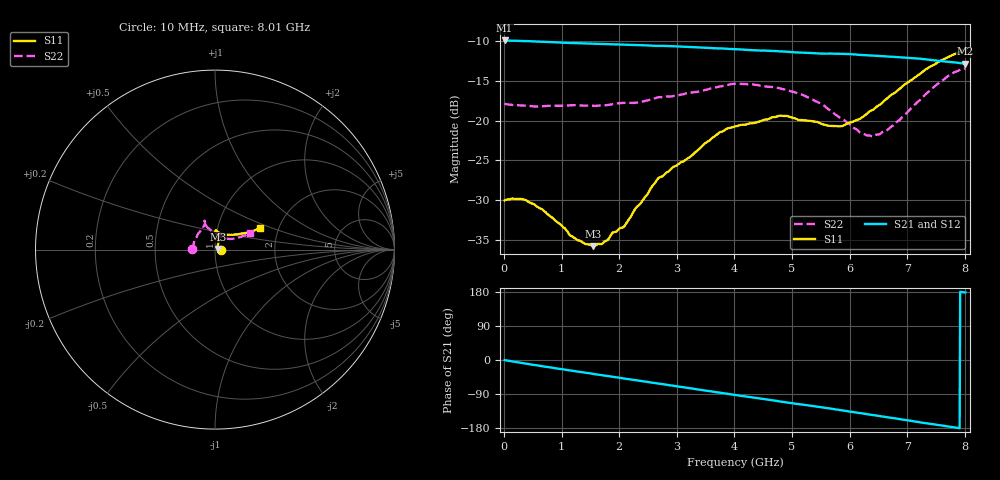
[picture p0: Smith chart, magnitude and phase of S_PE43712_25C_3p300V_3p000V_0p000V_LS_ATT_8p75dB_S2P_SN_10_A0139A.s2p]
! DEVICE ID: PE43712
! File Path: z:\PE43713\PE43713_CHAR_NOM_04292014\AMB\3p300\LS_ATT_8p75dB\PE43713_AMB_3p300V_3p000V_0p000V_LS_ATT_8p75dB_S2P_SN_10_A0139A.s2p
! Serial: 10
! Lot: A0139A
! Temp: 25C
! VDD: 3.300
! VSS: 0.000
! Control_Hi: 3.000
! Control_Lo: 0.000
! Attenuation Step: 8.75dB
! Port 1: RF1
! Port 2: RF2
! ThroughPath:1-2
! IDD: 0.0001466372
! ISS: -1.569e-007
#  Hz  S  RI  R  50
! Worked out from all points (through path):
!   801 points, 10 MHz to 8.01 GHz, reference 50 ohm
!   highest |S21| = -9.92 dB at 10 MHz (marker M1); lowest = -12.8 dB at 8.01 GHz (marker M2)
!   group delay of S21, straight-line fit = 62.5 ps
!   lowest |S11| = -35.8 dB at 1.54 GHz (marker M3), VSWR 1.03, Z = 51.6 + j0.428 ohm
!   |S11| at or under -10 dB: start of sweep to end of sweep
!   |S22| runs from -22.0 to -13.4 dB; largest |S21 - S12| = 0.0011
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1e7  0.0315 0.000124  0.3193 -0.00179  0.3192 -0.00174  -0.1274 0.000836
3e8  0.032 -0.00371  0.3142 -0.0422  0.3142 -0.0422  -0.1239 0.0135
5e8  0.0296 -0.00501  0.3076 -0.0684  0.3076 -0.0684  -0.1213 0.0213
9.6e8  0.0223 -0.00366  0.2846 -0.123  0.2848 -0.123  -0.1171 0.041
1.17e9  0.0188 -0.00133  0.2714 -0.1449  0.2715 -0.1451  -0.1144 0.0501
1.35e9  0.0173 0.000711  0.2593 -0.1631  0.2593 -0.1631  -0.1109 0.0566
1.54e9  0.0157 0.00415  0.2452 -0.181  0.2452 -0.1811  -0.1053 0.0653
1.72e9  0.015 0.00806  0.2308 -0.197  0.2308 -0.197  -0.101 0.0728
2.09e9  0.0139 0.0167  0.1979 -0.2265  0.1979 -0.2263  -0.0936 0.0891
2.68e9  0.0191 0.0391  0.138 -0.2609  0.138 -0.2609  -0.0705 0.1215
3.24e9  0.0153 0.0575  0.0756 -0.2801  0.0757 -0.2802  -0.0598 0.1372
3.72e9  0.0133 0.082  0.0219 -0.2838  0.0217 -0.2837  -0.0557 0.1534
4.01e9  0.00987 0.0915  -0.0104 -0.2814  -0.0104 -0.2813  -0.0588 0.16
4.79e9  0.00493 0.1075  -0.0901 -0.2573  -0.0901 -0.2576  -0.0561 0.1496
5.35e9  0.016 0.0978  -0.1387 -0.227  -0.1386 -0.2269  -0.0471 0.128
5.84e9  0.0366 0.0845  -0.1767 -0.1947  -0.1767 -0.1949  -0.0155 0.1026
6.28e9  0.0719 0.0818  -0.2042 -0.1573  -0.2038 -0.1573  0.0241 0.0777
6.42e9  0.0845 0.0823  -0.2111 -0.1451  -0.2108 -0.1451  0.0375 0.0705
6.68e9  0.1133 0.0841  -0.2222 -0.1203  -0.2219 -0.1205  0.0644 0.0615
7.55e9  0.2112 0.103  -0.2353 -0.0332  -0.235 -0.0332  0.1558 0.075
7.81e9  0.235 0.1138  -0.2324 -0.00965  -0.2323 -0.00974  0.1812 0.0863
8.01e9  0.2516 0.1215  -0.2278 0.007  -0.2275 0.00669  0.1925 0.0914
